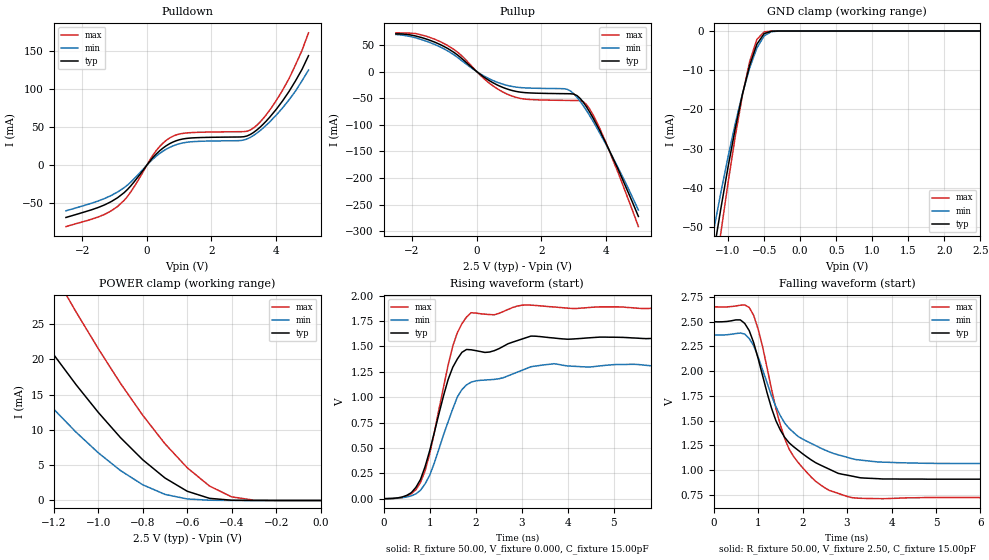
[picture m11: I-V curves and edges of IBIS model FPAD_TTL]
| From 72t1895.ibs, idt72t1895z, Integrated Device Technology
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|   Model FPAD_TTL
[Model]   FPAD_TTL
Model_type   3-state
Polarity   Non-Inverting
Enable   Active-Low
Vmeas =  1.250V
C_comp   3.00pF   NA   NA
[Temperature Range]   25.00   85.00   -40.00
[Voltage Range]   2.50V   2.30V   2.70V
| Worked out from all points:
|   slope of the pulldown table from 0 to 0.375 V, typ, clamps not added: 20.8 ohm
|   slope of the pullup table from 0 to 0.375 V, typ, clamps not added: 22.8 ohm
|   GND clamp passes 1 mA (typ) near -0.51 V on its own axis
|   POWER clamp passes 1 mA (typ) near -0.57 V on its own axis
|   rising waveform, R_fixture 50.00, V_fixture 0.000, C_fixture 15.00pF: 20-80 % time 580ps typ, 637ps min, 547ps max; typ from 0 V to 1.59 V
|   falling waveform, R_fixture 50.00, V_fixture 2.50, C_fixture 15.00pF: 20-80 % time 859ps typ, 922ps min, 758ps max; typ from 2.5 V to 0.91 V
[Pulldown]
| voltage   I(typ)   I(min)   I(max)
-2.5V     -68.7mA    -59.9mA    -80.7mA
-1.5V     -55.54mA   -46.94mA   -68mA
-900mV    -42.65mA   -35.17mA   -54.12mA
-500mV    -27.42mA   -22.41mA   -35.32mA
300mV     15.04mA    12.19mA    19.67mA
800mV     30.27mA    25.19mA    37.94mA
2.9V      37.11mA    32.42mA    44.04mA
3.3V      43.01mA    39.08mA    48.93mA
3.7V      58.35mA    52.83mA    66.66mA
4.2V      84.6mA     75.39mA    98.7mA
4.6V      111mA      97.59mA    132mA
5V        144mA      125mA      174mA
[Pullup]
| voltage   I(typ)   I(min)   I(max)
-2.5V     70.79mA    69.58mA    72.7mA
-1.7V     63.76mA    59.86mA    68.67mA
-900mV    43.46mA    38.9mA     48.97mA
-500mV    26.48mA    22.2mA     31.66mA
200mV     -9.353mA   -7.544mA   -11.93mA
1.1V      -35.64mA   -28.03mA   -46.18mA
2.8V      -41.57mA   -33.39mA   -54.16mA
3.1V      -45.1mA    -48.25mA   -54.37mA
3.3V      -57.93mA   -64.46mA   -56.63mA
3.5V      -76.66mA   -83.4mA    -70.99mA
3.8V      -110mA     -115mA     -106mA
5V        -272mA     -260mA     -291mA
[GND_clamp]
| voltage   I(typ)   I(min)   I(max)
-2.5V     -221mA     -196mA     -255mA
-1.2V     -56.53mA   -50.9mA    -64.94mA
-1.1V     -45.3mA    -41.22mA   -51.5mA
-1V       -34.68mA   -32.07mA   -38.72mA
-900mV    -24.85mA   -23.59mA   -26.87mA
-800mV    -16.08mA   -15.96mA   -16.35mA
-700mV    -8.721mA   -9.411mA   -7.76mA
-600mV    -3.357mA   -4.326mA   -2.135mA
-500mV    -667uA     -1.241mA   -218uA
-400mV    -58.99uA   -179uA     -9.374uA
-300mV    -2.618uA   -14.77uA   -139nA
2.5V      25.05nA    49.28nA    24.82nA
[POWER_clamp]
| voltage   I(typ)   I(min)   I(max)
-2.5V     85.21mA    68.62mA    107mA
-1.6V     39.45mA    28.25mA    55.23mA
-1.4V     29.75mA    20.21mA    43.52mA
-1.3V     25.1mA     16.46mA    37.78mA
-1.2V     20.64mA    12.93mA    32.17mA
-1.1V     16.41mA    9.679mA    26.72mA
-800mV    5.767mA    2.226mA    12.07mA
-600mV    1.308mA    217uA      4.638mA
-500mV    308uA      38.03uA    2.054mA
-400mV    34.83uA    4.694uA    512uA
-300mV    2.145uA    415nA      47.35uA
0V        25.05nA    25.08nA    27nA
[Ramp]
| variable   typ   min   max
dV/dt_r   0.96/0.33n   0.79/0.36n   1.14/0.34n
dV/dt_f   0.96/0.35n   0.82/0.35n   1.14/0.38n
R_load = 50.00
[Rising Waveform]
R_fixture = 50.00
V_fixture = 0.000
C_fixture = 15.00pF
R_dut = 0.75
L_dut = 8.10nH
C_dut = 0.53pF
| time   V(typ)   V(min)   V(max)
0s        0V         0V         0V
500ps     32.56mV    16.83mV    24.6mV
800ps     190mV      82.94mV    160mV
1ns       474mV      231mV      444mV
1.5ns     1.294V     884mV      1.502V
1.7ns     1.442V     1.075V     1.724V
1.9ns     1.467V     1.148V     1.832V
3.2ns     1.602V     1.3V       1.907V
3.7ns     1.583V     1.33V      1.889V
9.9ns     1.588V     1.31V      1.889V
[Falling Waveform]
R_fixture = 50.00
V_fixture = 2.50
C_fixture = 15.00pF
R_dut = 0.75
L_dut = 8.10nH
C_dut = 0.53pF
| time   V(typ)   V(min)   V(max)
0s        2.5V       2.366V     2.65V
600ps     2.518V     2.385V     2.666V
800ps     2.41V      2.33V      2.643V
1ns       2.129V     2.144V     2.426V
1.4ns     1.501V     1.642V     1.623V
1.7ns     1.276V     1.422V     1.211V
2.2ns     1.103V     1.27V      928mV
2.6ns     1.011V     1.186V     797mV
4.1ns     912mV      1.077V     717mV
9.9ns     910mV      1.068V     724mV
